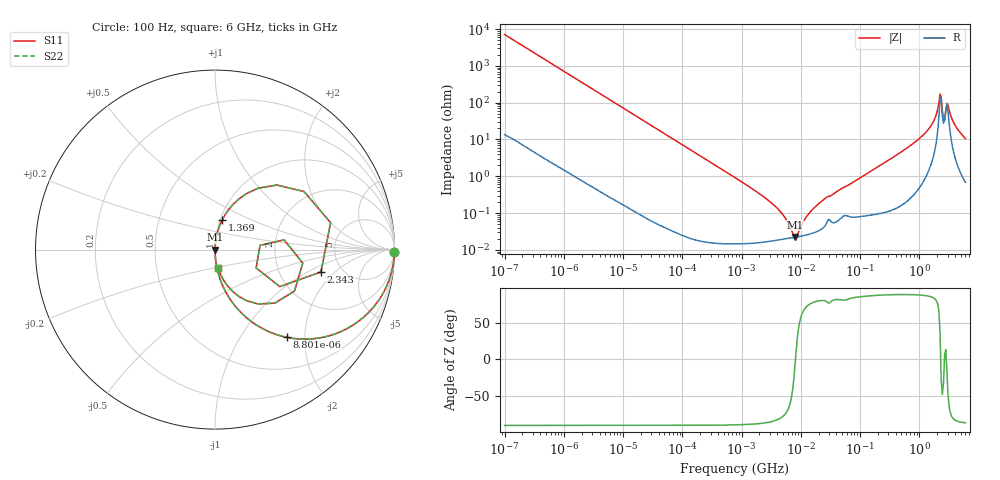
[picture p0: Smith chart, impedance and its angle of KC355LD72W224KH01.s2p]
!Murata Part Number: KC355LD72W224KH01
!These Parameters are Measured in Series Mode Connection
!Data Generated on Mar 13, 2026
!  o--ll--o
!Port1  Port2
!  o------o
!Operation Temp=25[degC], DC Bias Voltage=0[V]
!Freq. Start=100[Hz] Stop=6[GHz] 401[Steps]
# Hz S RI R 50
!Freq.(Hz) S11(Real) S11(Imag) S21(Real) S21(Imag) S12(Real) S12(Imag) S22(Real) S22(Imag)
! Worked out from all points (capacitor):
!   401 points, 100 Hz to 6 GHz, reference 50 ohm
!   read as one part in series: C = 223 nF near 109 Hz
!   lowest |Z| = 22.3 mohm at 7.948 MHz (marker M1)
!   series resonance near 8.123 MHz, so ESL is about 1.7 nH
!   S11 on the Smith chart (normalised r, x): 100 Hz: open; 8.801 kHz: 1.00, -1.63; 1.369 GHz: 1.02, +0.35; 2.343 GHz: 3.47, -1.36; 6 GHz: 1.01, -0.21
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100  0.9998 -0.014  0.000224 0.014  0.000224 0.014  0.9998 -0.014
2008  0.9265 -0.2599  0.0735 0.2599  0.0735 0.2599  0.9265 -0.2599
3931  0.768 -0.421  0.232 0.421  0.232 0.421  0.768 -0.421
8801  0.3991 -0.4886  0.6009 0.4886  0.6009 0.4886  0.3991 -0.4886
18016  0.1376 -0.3433  0.8624 0.3433  0.8624 0.3433  0.1376 -0.3433
40335  0.0312 -0.1725  0.9688 0.1725  0.9688 0.1725  0.0312 -0.1725
774597  0.00023 -0.00919  0.9998 0.00919  0.9998 0.00919  0.00023 -0.00919
3712478  0.000182 -0.00151  0.9998 0.00151  0.9998 0.00151  0.000182 -0.00151
5311619  0.000198 -0.000758  0.9998 0.000758  0.9998 0.000758  0.000198 -0.000758
7947587  0.000219 -3.71e-05  0.9998 3.71e-05  0.9998 3.71e-05  0.000219 -3.71e-05
1.555665e7  0.000283 0.00119  0.9997 -0.00119  0.9997 -0.00119  0.000283 0.00119
2.662322e7  0.000501 0.00256  0.9995 -0.00256  0.9995 -0.00256  0.000501 0.00256
3.124326e8  0.00192 0.0281  0.9981 -0.0281  0.9981 -0.0281  0.00192 0.0281
1.369159e9  0.0401 0.1655  0.9599 -0.1655  0.9599 -0.1655  0.0401 0.1655
1.95892e9  0.2431 0.3429  0.7569 -0.3429  0.7569 -0.3429  0.2431 0.3429
2.142435e9  0.4959 0.3236  0.5041 -0.3236  0.5041 -0.3236  0.4959 0.3236
2.34314e9  0.5903 -0.1245  0.4097 0.1245  0.4097 0.1245  0.5903 -0.1245
2.679998e9  0.251 0.0238  0.749 -0.0238  0.749 -0.0238  0.251 0.0238
3.065283e9  0.4426 -0.2313  0.5574 0.2313  0.5574 0.2313  0.4426 -0.2313
3.352442e9  0.2417 -0.3032  0.7583 0.3032  0.7583 0.3032  0.2417 -0.3032
4.009986e9  0.0821 -0.2164  0.9179 0.2164  0.9179 0.2164  0.0821 -0.2164
6e9  0.0176 -0.103  0.9824 0.103  0.9824 0.103  0.0176 -0.103
